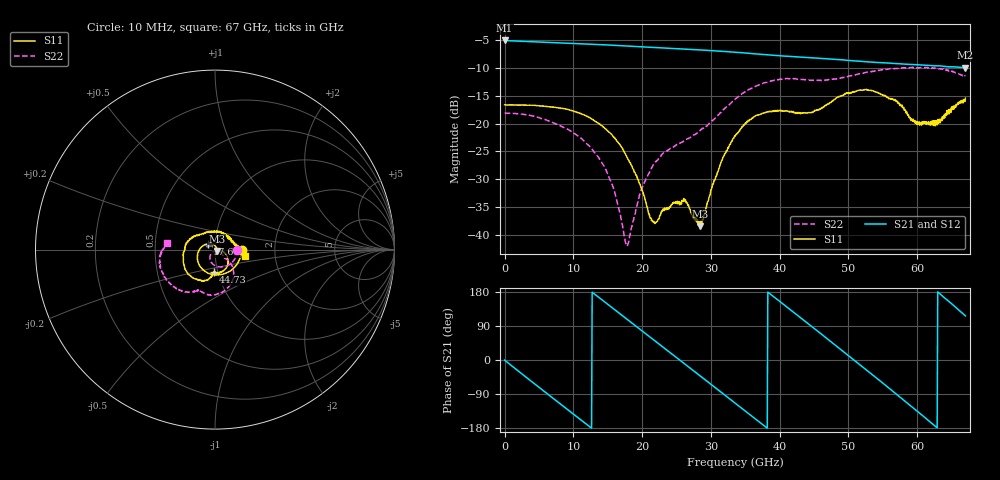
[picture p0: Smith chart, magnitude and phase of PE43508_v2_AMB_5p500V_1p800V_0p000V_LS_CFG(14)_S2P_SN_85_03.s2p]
!Keysight Technologies,N5227A,US51270237,A.10.43.00
!Date: Wednesday, August 22, 2018 17:07:59
!Correction: S11(Full 2 Port(1,3))
!S31(Full 2 Port(1,3))
!S13(Full 2 Port(1,3))
!S33(Full 2 Port(1,3))
!S2P File: Measurements: S11, S31, S13, S33:
# Hz S  dB  R 50
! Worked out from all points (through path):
!   801 points, 10 MHz to 67 GHz, reference 50 ohm
!   highest |S21| = -5.00 dB at 10 MHz (marker M1); lowest = -9.9 dB at 66.92 GHz (marker M2)
!   group delay of S21, straight-line fit = 39.6 ps
!   lowest |S11| = -38.5 dB at 28.4 GHz (marker M3), VSWR 1.02, Z = 50.9 - j0.77 ohm
!   |S11| at or under -10 dB: start of sweep to end of sweep
!   |S22| runs from -42.1 to -9.8 dB; largest |S21 - S12| = 0.003
!   S11 on the Smith chart (normalised r, x): 10 MHz: 1.35, -0.00; 17.68 GHz: 0.92, +0.06; 44.73 GHz: 0.95, -0.24; 67 GHz: 1.39, -0.10
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1e7  -16.60 -0.4  -5.00 -0.2  -5.00 -0.2  -18.11 -0.4
2.522125e9  -16.65 -32.9  -5.15 -36.7  -5.14 -36.7  -18.30 -26.9
5.70415e9  -16.85 -72.0  -5.31 -81.9  -5.31 -81.9  -19.17 -58.5
8.300012e9  -17.23 -102.9  -5.45 -118.6  -5.44 -118.6  -20.52 -82.7
1.123082e10  -18.27 -136.2  -5.61 -159.9  -5.60 -159.9  -22.73 -107.1
1.491528e10  -21.22 -179.6  -5.81 148.3  -5.81 148.3  -28.86 -130.9
1.767861e10  -25.77 144.0  -5.98 109.5  -5.98 109.5  -41.68 -94.2
2.127932e10  -37.03 50.2  -6.22 58.9  -6.21 58.9  -28.30 -27.7
2.236791e10  -37.24 -6.7  -6.30 43.6  -6.29 43.6  -26.38 -31.9
2.61361e10  -33.98 -82.1  -6.55 -9.3  -6.54 -9.3  -23.11 -42.5
2.839701e10  -38.49 -39.5  -6.70 -41.2  -6.70 -41.2  -21.27 -40.1
3.099288e10  -28.72 -11.9  -6.90 -78.0  -6.91 -77.9  -18.57 -41.3
3.3505e10  -22.28 -29.9  -7.12 -113.6  -7.12 -113.5  -15.62 -51.0
3.869672e10  -17.80 -73.3  -7.63 173.1  -7.63 173.2  -12.34 -80.8
4.196249e10  -17.82 -90.2  -7.93 127.0  -7.91 127.0  -11.88 -98.6
4.472582e10  -17.97 -93.8  -8.12 87.6  -8.11 87.6  -12.18 -108.6
5.033624e10  -14.39 -116.1  -8.64 6.7  -8.63 6.7  -11.37 -118.8
5.586291e10  -15.53 179.8  -9.08 -73.7  -9.07 -74.0  -10.14 -138.7
5.870999e10  -18.35 135.1  -9.30 -115.9  -9.32 -116.0  -9.97 -150.0
6.180828e10  -19.78 62.2  -9.53 -162.5  -9.56 -162.7  -9.98 -164.3
6.691626e10  -16.02 -11.0  -9.91 117.9  -9.96 118.1  -11.37 172.9
6.7e10  -15.41 -12.4  -9.90 116.5  -9.95 116.7  -11.43 171.8
